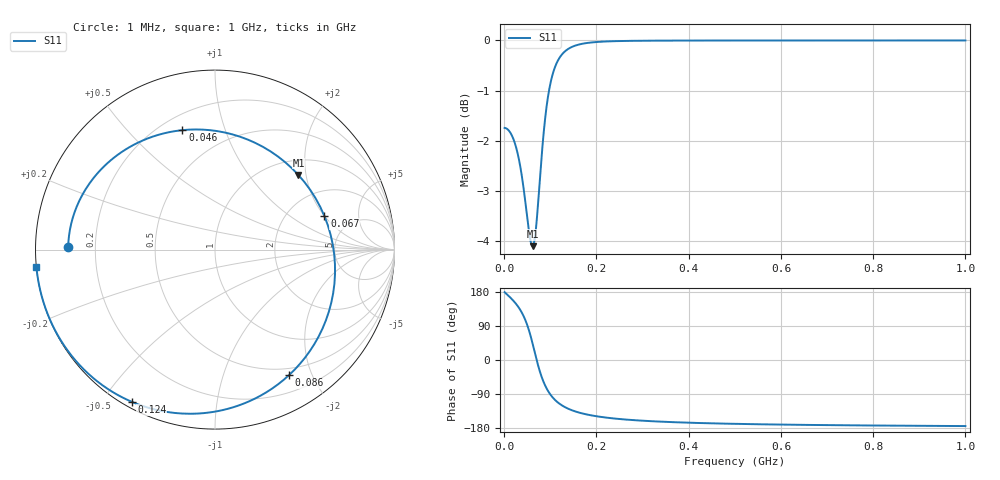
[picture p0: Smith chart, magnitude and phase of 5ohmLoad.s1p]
# MHz S RI R 50.0
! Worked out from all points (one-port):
!   999 points, 1 MHz to 1 GHz, reference 50 ohm
!   lowest |S11| = -4.1 dB at 62 MHz (marker M1), VSWR 4.31, Z = 66.6 + j90.6 ohm
!   |S11| at or under -10 dB: nowhere
!   S11 on the Smith chart (normalised r, x): 1 MHz: 0.10, +0.01; 46 MHz: 0.28, +0.72; 67 MHz: 3.17, +1.99; 86 MHz: 0.41, -1.68; 124 MHz: 0.02, -0.59; 1 GHz: 0.00, -0.05
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1  -0.818 0.0158
14  -0.7772 0.2224
26  -0.6617 0.417
36  -0.4788 0.5695
46  -0.1819 0.6655
54  0.1387 0.6293
58  0.309 0.5475
62  0.4651 0.4154
67  0.6096 0.1869
71  0.6642 -0.027
76  0.648 -0.2951
81  0.5537 -0.5261
86  0.4127 -0.6991
93  0.1925 -0.8443
100  -0.0113 -0.9045
111  -0.2632 -0.9051
124  -0.4648 -0.8476
126  -0.4888 -0.8369
145  -0.6549 -0.7348
170  -0.7735 -0.622
204  -0.8559 -0.5107
251  -0.9111 -0.4088
376  -0.9632 -0.2675
502  -0.9799 -0.1989
626  -0.9872 -0.1589
751  -0.9912 -0.1322
876  -0.9935 -0.1132
1000  -0.995 -0.0991
